PROGRAM MAIN
VAR
	FFU:FFU;
	tHeatbeat					:Ton;
	tON							:TON;
	bAdsCommErr					:BOOL;
	tOFF						:TON;
	
	//CE远程桌面开启
	bEnableCerDisp:BOOL;
	NT_StartProcess_Test:NT_StartProcess;
	
END_VAR

FFU();
IOMapping();
Interlock();


// PLC建立心跳
tHeatbeat(IN:=NOT tHeatbeat.Q , PT:=T#1S , Q=> , ET=> );
IF tHeatbeat.Q THEN
	GVL.stPLCtoPMC.bHeartBeatMonitor			:=NOT GVL.stPLCtoPMC.bHeartBeatMonitor;
END_IF

// PLC监控PMC心跳
IF GVL.stPMCtoPLC.bHeartBeatMonitor THEN
	tON(IN:=GVL.stPMCtoPLC.bHeartBeatMonitor , PT:=T#2S , Q=> , ET=> );
	tOFF(IN:=FALSE , PT:=T#2S , Q=> , ET=> );
	IF tON.Q THEN
		bAdsCommErr					:=TRUE;
	ELSE
		bAdsCommErr					:=FALSE;
	END_IF
ELSE
	tOFF(IN:=NOT GVL.stPMCtoPLC.bHeartBeatMonitor , PT:=T#2S , Q=> , ET=> );
	tON(IN:=FALSE , PT:=T#2S , Q=> , ET=> );
	IF tOFF.Q THEN
		bAdsCommErr					:=TRUE;
	ELSE
		bAdsCommErr					:=FALSE;
	END_IF
END_IF


//CE远程桌面开启
NT_StartProcess_Test(
	NETID:= ,
	PATHSTR:='\windows\CerDisp.exe' ,
	DIRNAME:='\windows' ,
	COMNDLINE:= , 
	START:=bEnableCerDisp ,
	TMOUT:= , 
	BUSY=> , 
	ERR=> , 
	ERRID=> );

END_PROGRAM
